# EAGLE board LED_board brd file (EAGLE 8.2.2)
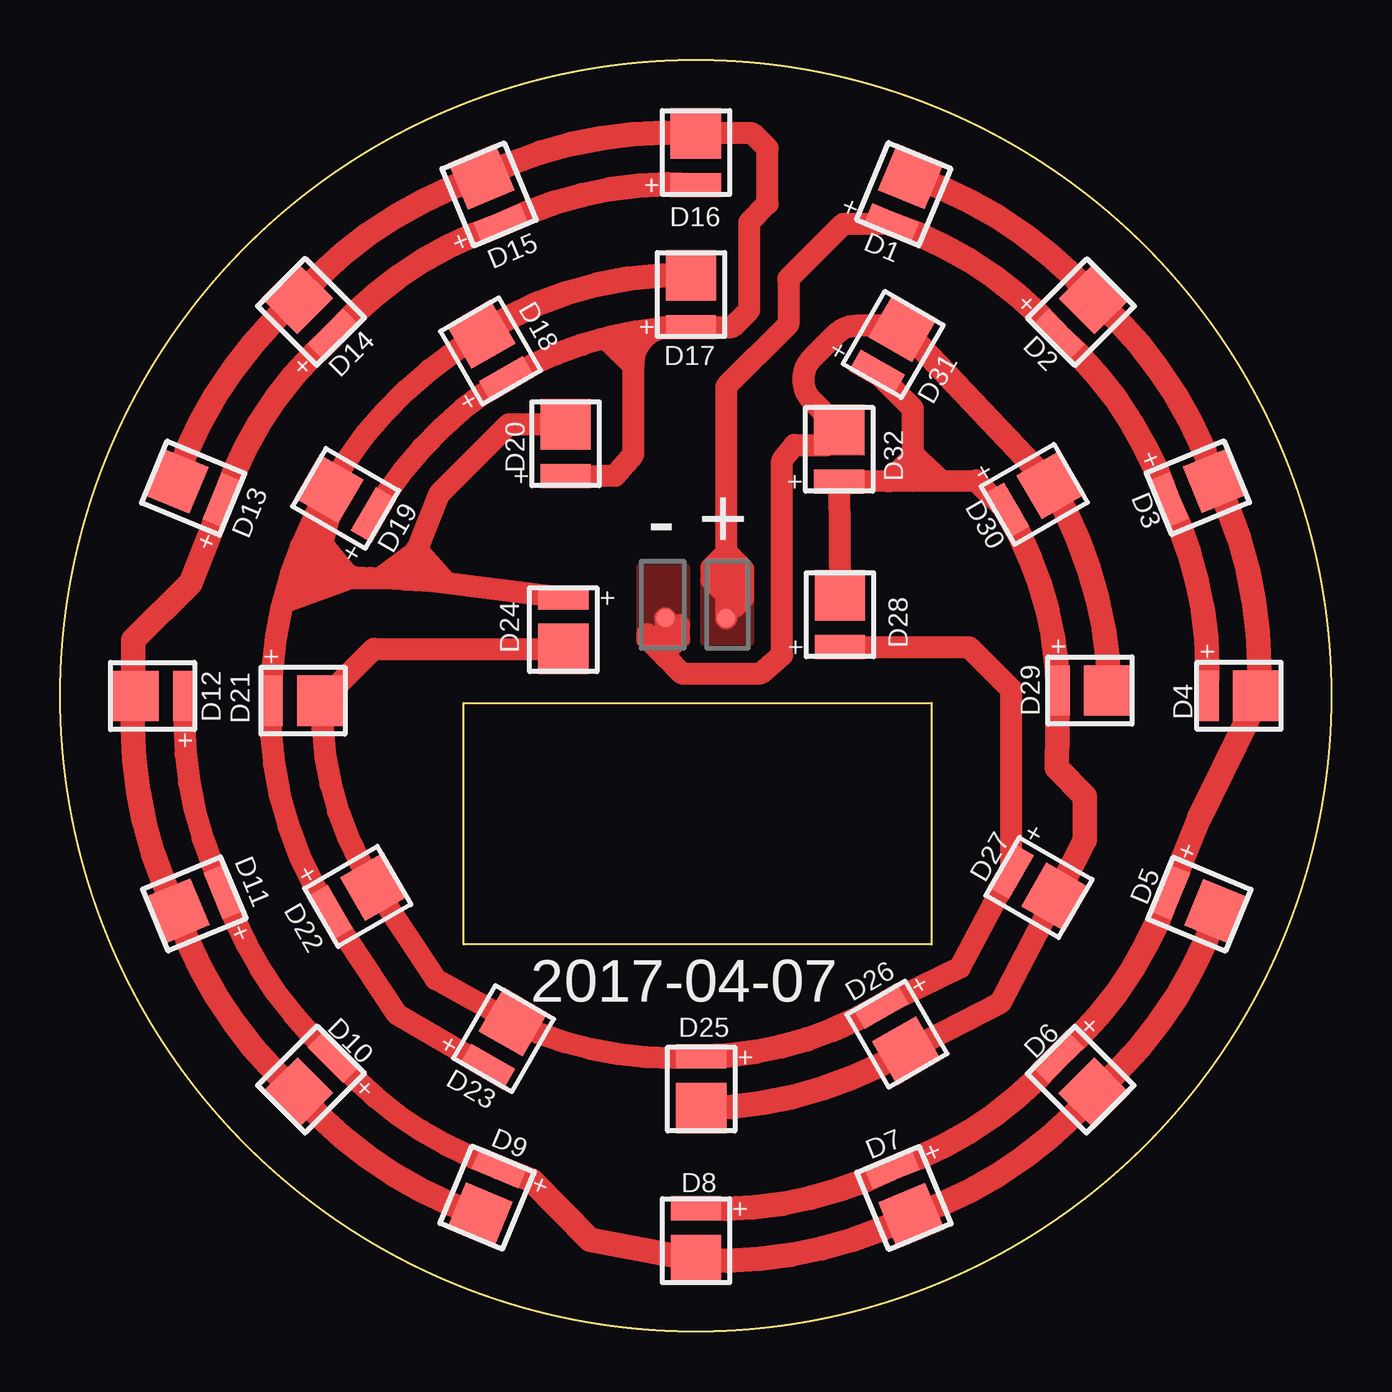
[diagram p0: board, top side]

Size 53 x 53 mm. Coordinates in mm from the lower left corner, seen from the top.
Outline: 36.33,16.14 16.83,16.14 16.83,26.21 36.33,26.21 36.33,16.14
Outline: circle at 26.5,26.5 radius 26.5
Copper layers (1*16): Top 0.035mm / dielectric 1.5mm / Bottom 0.035mm
Design rules "NOA Eagle Rule": minimum track width 7mil, minimum drill 12mil, track to track 7mil, track to pad 7mil, pad to pad 7mil, via to via 7mil, smd to smd 0mil, copper to edge 20mil, drill to drill 10mil, minimum pad ring 10mil, minimum via ring 6mil, stop-mask expansion 2mil, vias tented up to drill 25mil, thermal gap 10mil

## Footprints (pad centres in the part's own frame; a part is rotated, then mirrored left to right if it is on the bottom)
LED_2835 = smd 2.1 x 1: + 0,0.8 | smd 2.1 x 2.1: - 0,-1.35
1P-30MIL = smd 0.762 x 0.762: P$1 0,0

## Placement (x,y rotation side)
D1  [LED_2835]  34.95,46.9 157.5 top
D2  [LED_2835]  42.17,42.1 135 top
D3  [LED_2835]  46.92,34.96 112.5 top
D4  [LED_2835]  48.59,26.5 90 top
D5  [LED_2835]  46.98,18.02 67.5 top
D6  [LED_2835]  42.15,10.89 45 top
D7  [LED_2835]  34.97,6.07 22.5 top
D8  [LED_2835]  26.51,4.34 0 top
D9  [LED_2835]  18.02,6.09 337.5 top
D10  [LED_2835]  10.85,10.9 315 top
D11  [LED_2835]  6.11,18.03 292.5 top
D12  [LED_2835]  4.41,26.49 270 top
D13  [LED_2835]  6.06,34.94 247.5 top
D14  [LED_2835]  10.85,42.11 225 top
D15  [LED_2835]  18.09,46.89 202.5 top
D16  [LED_2835]  26.51,48.59 180 top
D17  [LED_2835]  26.3,42.67 180 top
D18  [LED_2835]  18.22,40.4 210 top
D19  [LED_2835]  12.38,34.45 240 top
D20  [LED_2835]  21.07,36.46 180 top
D21  [LED_2835]  9.58,26.3 90 top
D22  [LED_2835]  11.94,17.86 120 top
D23  [LED_2835]  18.21,11.73 150 top
D24  [LED_2835]  20.98,29.8 0 top
D25  [LED_2835]  26.73,10.66 0 top
D26  [LED_2835]  34.61,12.87 30 top
D27  [LED_2835]  40.33,18.78 60 top
D28  [LED_2835]  32.51,29.33 180 top
D29  [LED_2835]  42.38,26.72 90 top
D30  [LED_2835]  40.13,34.62 120 top
D31  [LED_2835]  34.45,40.66 150 top
D32  [LED_2835]  32.48,36.23 180 top
TS1  [1P-30MIL]  27.77,29.74 0 top
TS2  [1P-30MIL]  25.23,29.74 0 top

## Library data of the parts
D1-D32 = Discrete
TS1 TS2 = Connector

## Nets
+24: D1.+ D2.+ D3.+ D4.+ TS1.P$1
GND: D29.- D30.- D31.- D32.- TS2.P$1
N$1: D1.- D2.- D3.- D4.- D5.+ D6.+ D7.+ D8.+
N$4: D5.- D6.- D7.- D8.- D9.+ D10.+ D11.+ D12.+
N$9: D9.- D10.- D11.- D12.- D13.+ D14.+ D15.+ D16.+
N$13: D13.- D14.- D15.- D16.- D17.+ D18.+ D19.+ D20.+
N$17: D17.- D18.- D19.- D20.- D21.+ D22.+ D23.+ D24.+
N$21: D21.- D22.- D23.- D24.- D25.+ D26.+ D27.+ D28.+
N$25: D25.- D26.- D27.- D28.- D29.+ D30.+ D31.+ D32.+

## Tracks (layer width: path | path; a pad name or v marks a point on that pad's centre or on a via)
+24
  Top 0.914: D1.+ 32.64,46.16 30.36,43.88 30.36,41.97 27.77,39.38 TS1.P$1 | 27.76,32.87 27.76,32.49 28.47,31.77 28.47,30.56 28.12,30.2 | 27.76,33.12 27.76,32.44 27.15,31.83 27.15,31.34 27.51,30.99 27.56,30.99
  Top 1.016: D1.+ arc-30 D2.+ arc-30 D3.+ arc-30 D4.+
  pour Top (no thermals): 28.83,28.7 26.8,28.7 26.8,31.88 28.83,31.88
GND
  Top 0.914: D31.- 35.04,41.92 33.22,41.92 arc45 32.32,41.55 31.36,40.58 arc90 31.36,38.79 32.48,37.67 D32.- 32.48,37.43 32,36.96 30.61,36.96 30.1,36.32 30.1,28.19 29.21,27.43 25.91,27.43 25.23,28.11 TS2.P$1 | 25.5,27.86 24.49,28.88 24.49,29.06 | 25.35,28.45 25.81,28.91 25.81,29.44
  Top 1.016: D31.- D30.- arc-30 D29.-
  pour Top (no thermals): 26.16,28.7 24.13,28.7 24.13,31.88 26.16,31.88
N$1
  Top 1.016: D1.- arc-30 D2.- arc-30 D3.- arc-30 D4.- 49.48,25.49 47.48,21.37 D5.+ arc-30 D6.+ arc-30 D7.+ arc-30 D8.+
N$4
  Top 0.914: D12.+ arc30 D11.+ arc30 D10.+ arc30 D9.+
  Top 1.016: D5.- arc-30 D6.- arc-30 D7.- arc-30 D8.- 22.1,3.82 19.66,6.31 D9.+
N$9
  Top 1.016: D9.- arc-30 D10.- arc-30 D11.- arc-30 D12.- 3.06,28.82 5.44,31.2 D13.+ arc-30 D14.+ arc-30 D15.+ arc-30 D16.+
N$13
  Top 0.914: D17.+ 28.02,41.87 28.73,42.58 28.73,46.24 29.49,47 29.49,49.31 28.86,49.95 D16.- | D17.+ arc30 D18.+ arc30 D19.+ | D20.+ 22.71,35.67 23.14,35.67 23.91,36.56 23.91,40.32 | 23.91,40.32 arc-90 25.46,41.87 D17.+ | 22.5,41.35 22.78,41.35 23.9,40.23 23.91,40.24 23.91,40.32
  Top 1.016: D13.- arc-30 D14.- arc-30 D15.- arc-30 D16.-
N$17
  Top 0.914: D24.+ 15.53,31.28 14.38,31.34 | 14.38,31.34 12.95,31.42 | D23.+ 14.03,13.24 D22.+ arc-35 D21.+ arc-30 D19.- | D19.- arc-30 D18.- | 12.04,31.46 12.95,31.42 | 12.04,31.46 10.6,31.53 | 10.6,31.53 9.63,31.53 | 10.6,31.53 11.31,34.2 D19.- | D20.- 18.7,37.81 15.8,34.91 14.88,32.58 | 14.88,32.58 14.38,31.34 | 10.67,33.13 12.07,31.46 arc90 12.06,31.46 12.04,31.46 | 9.3,30.39 12.22,31.46 arc90 12.26,31.42 12.95,31.42 | 14.86,32.52 13.34,31.41 12.96,31.41 arc-90 12.95,31.42 | 16.03,31.28 14.86,32.6 arc-90 14.88,32.59 14.88,32.58
  Top 1.016: D17.- arc35 D18.-
N$21
  Top 0.914: D24.- 13.08,28.45 D21.- arc35 D22.- 15.65,14.69 D23.- arc30 D25.+ | D26.+ 37.52,15.18 D27.+ 39.64,26.78 37.89,28.53 D28.+
  Top 1.016: D25.+ arc30 D26.+
N$25
  Top 0.914: 35.54,35.45 D32.+ D28.- | 35.54,35.45 38.18,35.47 D30.+ | D31.+ 35.54,38.48 35.54,36.43 | 34.55,35.44 35.54,36.44 | 36.73,35.47 35.54,36.59 35.54,36.44 | 35.54,35.45 35.54,36.43 | 35.54,36.43 35.54,36.44 | D26.- 39.22,13.73 D27.-
  Top 1.016: D25.- arc30 D26.- | D27.- 42.73,20.48 42.73,22.31 41.56,23.48 D29.+ arc30 D30.+

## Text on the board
tPlace: - | + | 2017-04-07
tTest: 板厚1mm | 3K色温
